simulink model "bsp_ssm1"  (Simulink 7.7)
settings: Solver=ode45  StartTime=0  StopTime=10  FixedStep=0.1  RelTol=1e-3
libraries: simulink x2

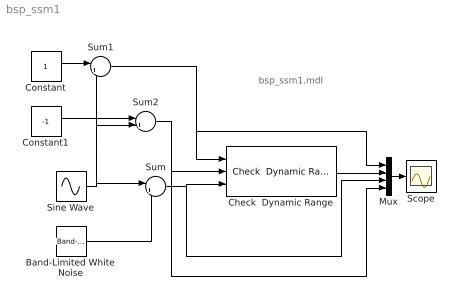
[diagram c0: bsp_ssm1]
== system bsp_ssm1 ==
  note: bsp_ssm1.mdl
  Band-Limited White Noise : simulink/Sources/Band-Limited White Noise  SystemSampleTime=-1  Cov=[0.001]  Ts=0.01  seed=[23341]
  Check  Dynamic Range : simulink/Model Verification/Check  Dynamic Range  Description=min < sig < max  SystemSampleTime=-1  enabled=on  stopWhenAssertionFail=off  export=on  icon=graphic
  Constant : Constant
  Constant1 : Constant  Value=-1
  Mux : Mux
  Scope : Scope
  Sine Wave : Sin  SampleTime=0
  Sum : Sum  Inputs=|++
  Sum1 : Sum  Inputs=|++
  Sum2 : Sum  Inputs=|++
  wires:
  Band-Limited White Noise/1 -> Sum/2
  Constant/1 -> Sum1/1
  Constant1/1 -> Sum2/1
  Sum1/1 -> Check  Dynamic Range/1, Mux/1
  Mux/1 -> Scope/1
  Sum/1 -> Check  Dynamic Range/3, Mux/3
  Sum2/1 -> Check  Dynamic Range/2, Mux/4
  Check  Dynamic Range/1 -> Mux/2
  Sine Wave/1 -> Sum/1, Sum1/2, Sum2/2
